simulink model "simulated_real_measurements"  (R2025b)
settings: Solver=VariableStepAuto  StartTime=0.0  StopTime=120  RelTol=1e-3
undefined symbols (not defined in the file): D, F, I, kp_pi, P, Ti_pi
libraries: simulink x5, slpidlib x2

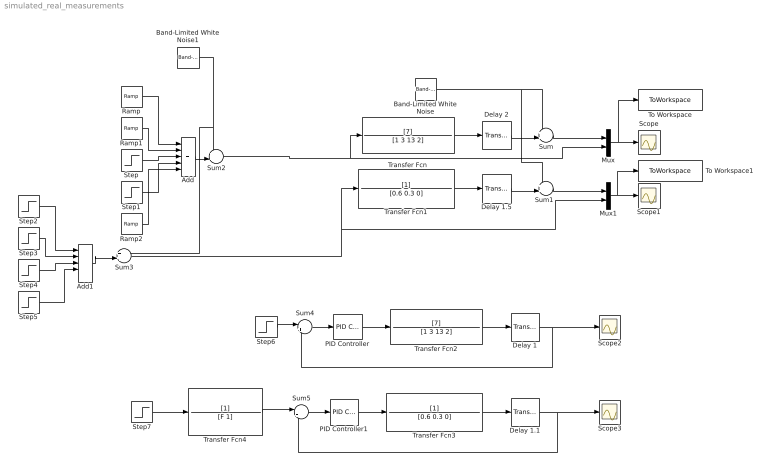
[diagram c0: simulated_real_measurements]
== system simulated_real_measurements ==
  Add : Sum  Inputs=+++++
  Add1 : Sum  Inputs=+++++
  Band-Limited White Noise : simulink/Sources/Band-Limited White Noise  Cov=[0.0003]  Ts=0.05  seed=[23341]
  Band-Limited White Noise1 : simulink/Sources/Band-Limited White Noise  Cov=[0.000003]  Ts=0.01  seed=[21371]
  Delay 1 : TransportDelay  DelayTime=2
  Delay 1.1 : TransportDelay  DelayTime=1.5
  Delay 1.5 : TransportDelay  DelayTime=1.5
  Delay 2 : TransportDelay  DelayTime=2
  Mux : Mux  Inputs=2
  Mux1 : Mux  Inputs=2
  PID Controller : slpidlib/PID Controller  Controller=PI  Form=Ideal  TimeDomain=Continuous-time  UseExternalTs=off  SampleTime=-1  IntegratorMethod=Forward Euler  FilterMethod=Forward Euler  ControllerParametersSource=internal  P=kp_pi*0.36  I=1/Ti_pi  UseKiTs=off  D=0  UseExternalDerivativeSource=off  N=100  UseFilter=on  TunerSelectOption=Transfer Function Based (PID Tuner App)  InitialConditionSource=internal  InitialConditionForIntegrator=0  InitialConditionForFilter=0  DifferentiatorICPrevScaledInput=0  ExternalReset=none  TrackingMode=off  Kt=1  LimitOutput=off  SatLimitsSource=internal  UpperSaturationLimit=inf  LowerSaturationLimit=-inf  LinearizeAsGain=on  AntiWindupMode=none  Kb=1  LimitIntegrator=off  UpperIntegratorSaturationLimit=inf  LowerIntegratorSaturationLimit=-inf  POutMin=[]  POutMax=[]  IOutMin=[]  IOutMax=[]  DOutMin=[]  DOutMax=[]  NOutMin=[]  NOutMax=[]  SumOutMin=[]  SumOutMax=[]  SaturationOutMin=[]  SaturationOutMax=[]  PParamMin=[]  PParamMax=[]  IParamMin=[]  IParamMax=[]  DParamMin=[]  DParamMax=[]  NParamMin=[]  NParamMax=[]  KbParamMin=[]  KbParamMax=[]  KtParamMin=[]  KtParamMax=[]  KbOutMin=[]  KbOutMax=[]  KtOutMin=[]  KtOutMax=[]  IntegratorOutMin=[]  IntegratorOutMax=[]  FilterOutMin=[]  FilterOutMax=[]  SumI1OutMin=[]  SumI1OutMax=[]  SumI2OutMin=[]  SumI2OutMax=[]  SumI3OutMin=[]  SumI3OutMax=[]  SumI4OutMin=[]  SumI4OutMax=[]  SumDOutMin=[]  SumDOutMax=[]  DifferentiatorOutMin=[]  DifferentiatorOutMax=[]  FilterDiffOutCoefMin=[]  FilterDiffOutCoefMax=[]  ReciprocalOutMin=[]  ReciprocalOutMax=[]  SumDenOutMin=[]  SumDenOutMax=[]  SumNumOutMin=[]  SumNumOutMax=[]  DivideOutMin=[]  DivideOutMax=[]  UdiffTsProdOutMin=[]  UdiffTsProdOutMax=[]  NTsProdOutMin=[]  NTsProdOutMax=[]  UintegralTsProdOutMin=[]  UintegralTsProdOutMax=[]  UngainTsProdOutMin=[]  UngainTsProdOutMax=[]  ClampingZeroOutDataTypeStr=Inherit: Inherit via back propagation  ClampingZeroOutMin=[]  ClampingZeroOutMax=[]  FilterDenConstantOutDataTypeStr=Inherit: Inherit via back propagation  FilterDenConstantOutMin=[]  FilterDenConstantOutMax=[]  PCopyOutDataTypeStr=Inherit: Inherit via back propagation  PCopyOutMin=[]  PCopyOutMax=[]  NCopyOutDataTypeStr=Inherit: Inherit via back propagation  NCopyOutMin=[]  NCopyOutMax=[]  IntegratorContinuousStateAttributes=''  IntegratorStateMustResolveToSignalObject=off  IntegratorRTWStateStorageClass=Auto  FilterContinuousStateAttributes=''  FilterStateMustResolveToSignalObject=off  FilterRTWStateStorageClass=Auto  ParallelPVariant=Passthrough  IdealPVariant=InternalParameters  IVariant=InternalParameters  DVariant=Disabled  IntegratorVariant=Continuous  SatVariant=Disabled  AWVariant=Passthrough  PCopyVariant=Disabled  TRVariant=Disabled  FdbkBlocksVariant=Forward  IdealPFdbkVariant=Disabled  SatFdbkVariant=Disabled  DerivativeFilterVariant=Disabled  NVariant=Disabled  NCopyVariant=Disabled_SignalSpec  FilterICVariant=Disabled  IntegratorICVariant=InternalICs  ExternalResetVariant=Disabled  TRSumVariant=Passthrough  SumFdbkVariant=Disabled  SumVariant=Sum_PI  TsampFilterVariant=InternalTs  TsampNgainVariant=Passthrough  TsampIntegralVariant=Disabled_SignalSpec  ExternalSaturationOutDataTypeStr=Inherit: Same as second input  DerivativeSourceVariant=Disabled  PreIntVariant=InternalPreInt
  PID Controller1 : slpidlib/PID Controller  Controller=PID  Form=Parallel  TimeDomain=Continuous-time  UseExternalTs=off  SampleTime=-1  IntegratorMethod=Forward Euler  FilterMethod=Forward Euler  ControllerParametersSource=internal  P=P  I=I  UseKiTs=off  D=D  UseExternalDerivativeSource=off  N=100  UseFilter=on  TunerSelectOption=Transfer Function Based (PID Tuner App)  InitialConditionSource=internal  InitialConditionForIntegrator=0  InitialConditionForFilter=0  DifferentiatorICPrevScaledInput=0  ExternalReset=none  TrackingMode=off  Kt=1  LimitOutput=off  SatLimitsSource=internal  UpperSaturationLimit=inf  LowerSaturationLimit=-inf  LinearizeAsGain=on  AntiWindupMode=none  Kb=1  LimitIntegrator=off  UpperIntegratorSaturationLimit=inf  LowerIntegratorSaturationLimit=-inf  POutMin=[]  POutMax=[]  IOutMin=[]  IOutMax=[]  DOutMin=[]  DOutMax=[]  NOutMin=[]  NOutMax=[]  SumOutMin=[]  SumOutMax=[]  SaturationOutMin=[]  SaturationOutMax=[]  PParamMin=[]  PParamMax=[]  IParamMin=[]  IParamMax=[]  DParamMin=[]  DParamMax=[]  NParamMin=[]  NParamMax=[]  KbParamMin=[]  KbParamMax=[]  KtParamMin=[]  KtParamMax=[]  KbOutMin=[]  KbOutMax=[]  KtOutMin=[]  KtOutMax=[]  IntegratorOutMin=[]  IntegratorOutMax=[]  FilterOutMin=[]  FilterOutMax=[]  SumI1OutMin=[]  SumI1OutMax=[]  SumI2OutMin=[]  SumI2OutMax=[]  SumI3OutMin=[]  SumI3OutMax=[]  SumI4OutMin=[]  SumI4OutMax=[]  SumDOutMin=[]  SumDOutMax=[]  DifferentiatorOutMin=[]  DifferentiatorOutMax=[]  FilterDiffOutCoefMin=[]  FilterDiffOutCoefMax=[]  ReciprocalOutMin=[]  ReciprocalOutMax=[]  SumDenOutMin=[]  SumDenOutMax=[]  SumNumOutMin=[]  SumNumOutMax=[]  DivideOutMin=[]  DivideOutMax=[]  UdiffTsProdOutMin=[]  UdiffTsProdOutMax=[]  NTsProdOutMin=[]  NTsProdOutMax=[]  UintegralTsProdOutMin=[]  UintegralTsProdOutMax=[]  UngainTsProdOutMin=[]  UngainTsProdOutMax=[]  ClampingZeroOutDataTypeStr=Inherit: Inherit via back propagation  ClampingZeroOutMin=[]  ClampingZeroOutMax=[]  FilterDenConstantOutDataTypeStr=Inherit: Inherit via back propagation  FilterDenConstantOutMin=[]  FilterDenConstantOutMax=[]  PCopyOutDataTypeStr=Inherit: Inherit via back propagation  PCopyOutMin=[]  PCopyOutMax=[]  NCopyOutDataTypeStr=Inherit: Inherit via back propagation  NCopyOutMin=[]  NCopyOutMax=[]  IntegratorContinuousStateAttributes=''  IntegratorStateMustResolveToSignalObject=off  IntegratorRTWStateStorageClass=Auto  FilterContinuousStateAttributes=''  FilterStateMustResolveToSignalObject=off  FilterRTWStateStorageClass=Auto  ParallelPVariant=InternalParameters  IdealPVariant=Disabled  IVariant=InternalParameters  DVariant=InternalParameters  IntegratorVariant=Continuous  SatVariant=Disabled  AWVariant=Passthrough  PCopyVariant=Disabled  TRVariant=Disabled  FdbkBlocksVariant=Forward  IdealPFdbkVariant=Disabled  SatFdbkVariant=Disabled  DerivativeFilterVariant=ContFilter  NVariant=InternalParameters  NCopyVariant=Disabled  FilterICVariant=InternalICsFilter  IntegratorICVariant=InternalICs  ExternalResetVariant=Disabled  TRSumVariant=Passthrough  SumFdbkVariant=Disabled  SumVariant=Sum_PID  TsampFilterVariant=InternalTs  TsampNgainVariant=Passthrough  TsampIntegralVariant=Disabled_SignalSpec  ExternalSaturationOutDataTypeStr=Inherit: Same as second input  DerivativeSourceVariant=ErrorSignal  PreIntVariant=InternalPreInt
  Ramp : simulink/Sources/Ramp  slope=0.3  start=0  InitialOutput=0
  Ramp1 : simulink/Sources/Ramp  slope=-0.3  start=10  InitialOutput=0
  Ramp2 : simulink/Sources/Ramp  slope=0.3  start=100  InitialOutput=9.3
  Scope{,1..3} (4 alike) : Scope
  Step : Step  Time=45  Before=3  After=3.3  SampleTime=0
  Step1 : Step  Time=80  Before=3.3  After=3  SampleTime=0
  Step2 : Step  Time=0  After=0.5  SampleTime=0
  Step3 : Step  Time=10  Before=0.5  After=-0.5  SampleTime=0
  Step4 : Step  Time=30  Before=-0.1  After=0.1  SampleTime=0
  Step5 : Step  Time=80  Before=0.1  After=-0.1  SampleTime=0
  Step6 : Step  Time=0  After=0.3  SampleTime=0
  Step7 : Step  Time=0  After=0.3  SampleTime=0
  Sum{,1..3} (4 alike) : Sum  Inputs=++|
  Sum4 : Sum  Inputs=|+-
  Sum5 : Sum  Inputs=|+-
  To Workspace : ToWorkspace  VariableName=object_1  SaveFormat=Timeseries  SampleTime=0.1
  To Workspace1 : ToWorkspace  VariableName=object_2  SaveFormat=Timeseries  SampleTime=0.1
  Transfer Fcn : TransferFcn  Numerator=[7]  Denominator=[1 3 13 2]
  Transfer Fcn1 : TransferFcn  Denominator=[0.6 0.3 0]
  Transfer Fcn2 : TransferFcn  Numerator=[7]  Denominator=[1 3 13 2]
  Transfer Fcn3 : TransferFcn  Denominator=[0.6 0.3 0]
  Transfer Fcn4 : TransferFcn  Denominator=[F 1]
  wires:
  Sum/1 -> Mux/1
  Sum1/1 -> Mux1/1
  Add/1 -> Sum2/2
  Transfer Fcn/1 -> Delay 2/1
  Delay 2/1 -> Sum/2
  Transfer Fcn1/1 -> Delay 1.5/1
  Delay 1.5/1 -> Sum1/2
  Ramp/1 -> Add/1
  Ramp1/1 -> Add/2
  Step/1 -> Add/3
  Step1/1 -> Add/4
  Ramp2/1 -> Add/5
  Add1/1 -> Sum3/2
  Step2/1 -> Add1/1
  Step3/1 -> Add1/2
  Step4/1 -> Add1/3
  Step5/1 -> Add1/4
  Band-Limited White Noise/1 -> Sum1/1, Sum/1
  Mux/1 -> To Workspace/1, Scope/1
  Mux1/1 -> To Workspace1/1, Scope1/1
  Sum2/1 -> Transfer Fcn/1, Mux/2
  Band-Limited White Noise1/1 -> Sum3/1, Sum2/1
  Sum3/1 -> Mux1/2, Transfer Fcn1/1
  Transfer Fcn2/1 -> Delay 1/1
  PID Controller/1 -> Transfer Fcn2/1
  Step6/1 -> Sum4/1
  Sum4/1 -> PID Controller/1
  Delay 1/1 -> Scope2/1, Sum4/2
  Transfer Fcn3/1 -> Delay 1.1/1
  Delay 1.1/1 -> Sum5/2, Scope3/1
  Sum5/1 -> PID Controller1/1
  PID Controller1/1 -> Transfer Fcn3/1
  Step7/1 -> Transfer Fcn4/1
  Transfer Fcn4/1 -> Sum5/1
